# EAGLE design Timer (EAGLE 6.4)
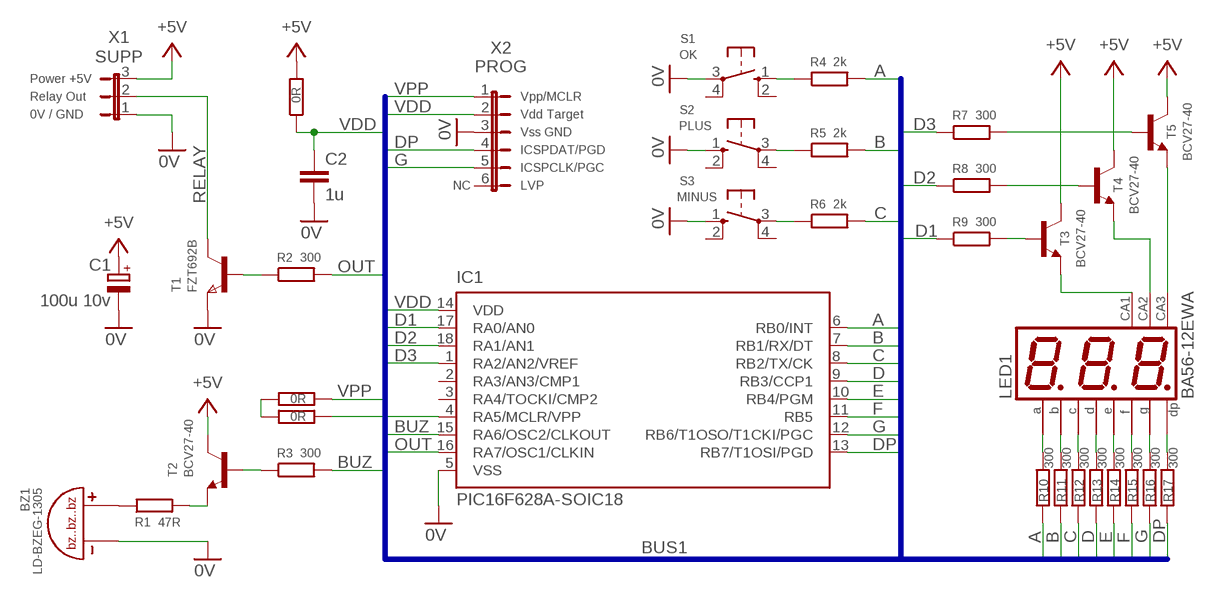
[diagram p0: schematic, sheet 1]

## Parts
BZ1  LD-BZEG-1305  LD-BZEG-1305LOUDITY  [LD-BZEG-1305]
C1  100u 10v  CPOL-EUSMCD  [SMC_D]
C2  1u  C-EUC1206K  [C1206K]
IC1  PIC16F628A-SOIC18  PIC16F628SO  [SO-18W]
J1  0R  R-EU_1206  [RESC3216X71N]
J2  0R  R-EU_1206  [RESC3216X71N]
J3  0R  R-EU_1206  [RESC3216X71N]
LED1  BA56-12EWA  [BX56-12]
R1  47R  R-EU_1206  [RESC3216X71N]
R2  300  R-EU_1206  [RESC3216X71N]
R3  300  R-EU_1206  [RESC3216X71N]
R4  2k  R-EU_1206  [RESC3216X71N]
R5  2k  R-EU_1206  [RESC3216X71N]
R6  2k  R-EU_1206  [RESC3216X71N]
R7  300  R-EU_1206  [RESC3216X71N]
R8  300  R-EU_1206  [RESC3216X71N]
R9  300  R-EU_1206  [RESC3216X71N]
R10  300  R-EU_1206  [RESC3216X71N]
R11  300  R-EU_1206  [RESC3216X71N]
R12  300  R-EU_1206  [RESC3216X71N]
R13  300  R-EU_1206  [RESC3216X71N]
R14  300  R-EU_1206  [RESC3216X71N]
R15  300  R-EU_1206  [RESC3216X71N]
R16  300  R-EU_1206  [RESC3216X71N]
R17  300  R-EU_1206  [RESC3216X71N]
S1  OK  10-XX  [B3F-10XX]
S2  PLUS  10-XX  [B3F-10XX]
S3  MINUS  10-XX  [B3F-10XX]
T1  FZT692B  NPNSOT223  [SOT223]
T2  BCV27-40  -NPN-SOT23_BEC  [SOT23-EBC]
T3  BCV27-40  -NPN-SOT23_BEC  [SOT23-EBC]
T4  BCV27-40  -NPN-SOT23_BEC  [SOT23-EBC]
T5  BCV27-40  -NPN-SOT23_BEC  [SOT23-EBC]
X1  SUPP  JP2W  [JP2W]
X2  PROG  JP6W  [JP6W]

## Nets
0V: BZ1.P$2 C1.- C2.2 IC1.5(VSS) S1.3(P) S2.1(S) S3.1(S) T1.3(E) X1.1 X2.3
+5V: C1.+ J1.2 T2.C T3.C T4.C T5.C X1.3
A: IC1.6(RB0/INT) R4.2 R10.1
B: IC1.7(RB1/RX/DT) R5.2 R11.1
BUZ: IC1.15(RA6/OSC2/CLKOUT) R3.2
C: IC1.8(RB2/TX/CK) R6.2 R12.1
D: IC1.9(RB3/CCP1) R13.1
D1: IC1.17(RA0/AN0) R9.1
D2: IC1.18(RA1/AN1) R8.1
D3: IC1.1(RA2/AN2/VREF) R7.1
DP: IC1.13(RB7/T1OSI/PGD) R17.1 X2.4
E: IC1.10(RB4/PGM) R14.1
F: IC1.11(RB5) R15.1
G: IC1.12(RB6/T1OSO/T1CKI/PGC) R16.1 X2.5
N$1: LED1.11(A) R10.2
N$2: LED1.7(B) R11.2
N$3: LED1.4(C) R12.2
N$4: LED1.2(D) R13.2
N$5: LED1.1(E) R14.2
N$6: LED1.10(F) R15.2
N$7: LED1.5(G) R16.2
N$8: LED1.3(DP) R17.2
N$9: LED1.12(CA) T3.B(E)
N$10: LED1.9(CA) T4.B(E)
N$11: LED1.8(CA) T5.B(E)
N$12: R9.2 T3.E(B)
N$13: R8.2 T4.E(B)
N$14: R7.2 T5.E(B)
N$15: R4.1 S1.1(S)
N$16: R5.1 S2.3(P)
N$17: R6.1 S3.3(P)
N$18: R2.1 T1.1(B)
N$19: R3.1 T2.E(B)
N$20: BZ1.P$1 R1.1
N$21: R1.2 T2.B(E)
N$23: J2.1 J3.1
OUT: IC1.16(RA7/OSC1/CLKIN) R2.2
RELAY: T1.2(C) T1.4(C) X1.2
VDD: C2.1 IC1.14(VDD) J1.1 X2.2
VPP: J3.2 X2.1
VPP': IC1.4(RA5/MCLR/VPP) J2.2
Unconnected: IC1.2(RA3/AN3/CMP1) IC1.3(RA4/TOCKI/CMP2) S1.2(S1) S1.4(P1) S2.2(S1) S2.4(P1) S3.2(S1) S3.4(P1) X2.6

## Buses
BUS1

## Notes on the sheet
- Power +5V
- Relay Out | Vpp/MCLR
- 0V / GND | Vdd Target
- Vss GND
- ICSPDAT/PGD
- ICSPCLK/PGC
- NC | LVP

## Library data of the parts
BZ1 = Timer:LD-BZEG-1305
C1 = Timer:CPOL-EU: POLARIZED CAPACITOR, European symbol
C2 = Timer:C-EU: CAPACITOR, European symbol
IC1 = Timer:PIC16F62*: FLASH-Based 8-Bit CMOS Microcontroller Source: http://ww1.microchip.com/downloads/en/DeviceDoc/40300C.pdf; MF: MICROCHIP; MPN: PIC16F628-20I/SO; OC_FARNELL: 9760415; OC_NEWARK: 23C4986
J1-J3 R1-R17 = Timer:R-EU_: RESISTOR, European symbol
LED1 = Timer:B?56-12*WA: 14.22mm (0.56INCH) THREE DIGIT NUMERIC DISPLAY Source: http://www.kingbright.com .. BA56-11EWA(Ver1189474895.pdf; OC_FARNELL: unknown; OC_NEWARK: unknown
S1-S3 = Timer:10-XX: OMRON SWITCH; MPN: B3F-1000; OC_FARNELL: 176432; OC_NEWARK: 36M3542
T1 = Timer:NPNSOT223: NPN TRANSISTOR; MPN: DJT4031N-13; OC_FARNELL: 1710672; OC_NEWARK: 25R4490
T2-T5 = Timer:*-NPN-: NPN Transistror
X1 = Timer:JP2W: JUMPER
X2 = Timer:JP6W

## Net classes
0 default: width 0.305 mm, drill 0.508 mm, clearance 0.305 mm

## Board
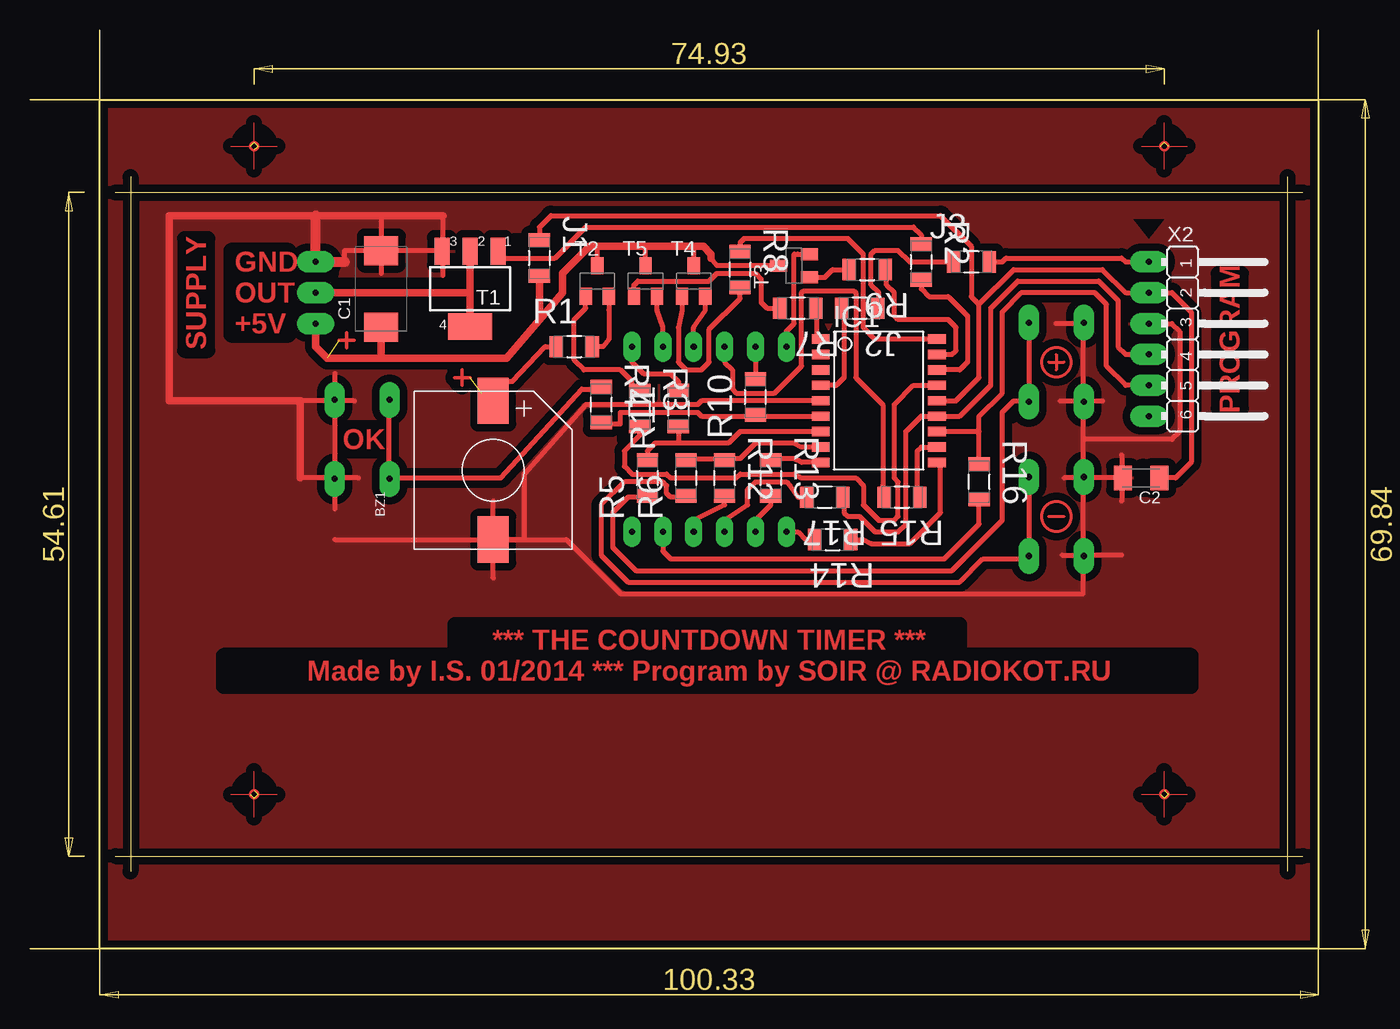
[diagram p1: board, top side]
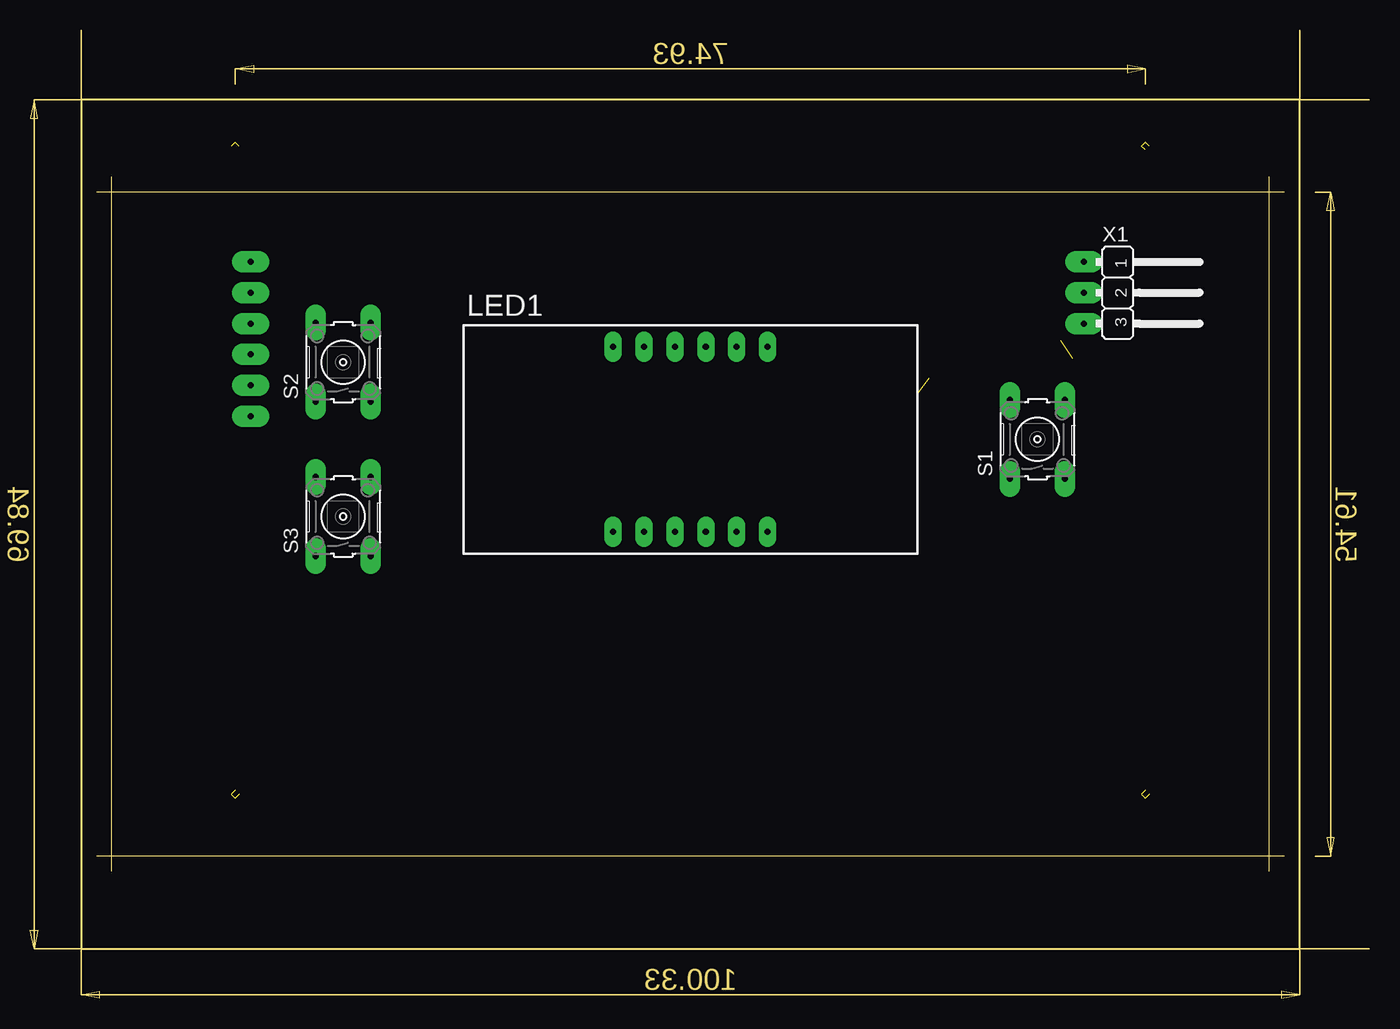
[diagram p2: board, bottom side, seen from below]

Size 110.21 x 79.67 mm. Coordinates in mm from the lower left corner, seen from the top.
Outline: 103.5,10.46 103.5,67.61
Outline: 8.25,67.61 8.25,10.46
Outline: 6.98,11.73 104.75,11.73
Outline: 6.98,66.34 104.75,66.34
Outline: 5.71,4.11 5.71,73.96 106.05,73.96 106.05,4.11 5.71,4.11
Copper layers (1*2): Top 0.035mm / dielectric 1.5mm / Route2 0.035mm
Design rules "default *": minimum track width 12mil, minimum drill 20mil, track to track 12mil, track to pad 12mil, pad to pad 12mil, via to via 12mil, smd to smd 12mil, copper to edge 20mil, drill to drill 40mil, minimum pad ring 10mil, minimum via ring 8mil, stop-mask expansion 6mil, vias tented up to drill 0mil, thermal gap 24mil
tRestrict: area 50.5,37.1 to 51.1,39.7; area 53,37.1 to 53.7,39.7; area 55.6,37.1 to 56.2,39.7; area 58.1,37.1 to 58.7,39.7; area 60.6,37.1 to 61.3,39.7; area 60.6,52.4 to 61.3,54.9; area 58.1,52.4 to 58.7,54.9; area 55.6,52.4 to 56.2,54.9; area 53,52.4 to 53.7,54.9; area 50.5,52.4 to 51.1,54.9; area 90.8,48.9 to 93.3,49.5; area 90.8,51.4 to 93.3,52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

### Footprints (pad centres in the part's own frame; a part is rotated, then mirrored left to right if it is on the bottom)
LD-BZEG-1305 = smd 2.54 x 3.81: P$1 0,5.715; P$2 0,-5.715
SMC_D = smd 2.4 x 2.8: + -3.15,0; - 3.15,0
C1206K = smd 1.5 x 2: 1 -1.5,0; 2 1.5,0
SO-18W = smd 0.762 x 1.46: 1 -5.08,-4.788; 2 -3.81,-4.788; 3 -2.54,-4.788; 4 -1.27,-4.788; 5 0,-4.788; 6 1.27,-4.788; 7 2.54,-4.788; 8 3.81,-4.788; 9 5.08,-4.788; 10 5.08,4.788; 11 3.81,4.788; 12 2.54,4.788; 13 1.27,4.788; 14 0,4.788; 15 -1.27,4.788; 16 -2.54,4.788; 17 -3.81,4.788; 18 -5.08,4.788
RESC3216X71N = smd 1.118 x 1.753: 1 -1.473,0; 2 1.473,0
BX56-12 = drill 0.5 pad 1.422 long: 1 -6.35,-7.62; 2 -3.81,-7.62; 3 -1.27,-7.62; 4 1.27,-7.62; 5 3.81,-7.62; 6 6.35,-7.62; 7 6.35,7.62; 8 3.81,7.62; 9 1.27,7.62; 10 -1.27,7.62; 11 -3.81,7.62; 12 -6.35,7.62
B3F-10XX = drill 0.5 pad 1.7 long: 1 -3.251,2.261; 2 3.251,2.261; 3 -3.251,-2.261; 4 3.251,-2.261
SOT223 = smd 1.219 x 2.235: 1 -2.311,-3.099; 2 0,-3.099; 3 2.311,-3.099 | smd 3.6 x 2.2: 4 0,3.099
SOT23-EBC = smd 1 x 1.4: B 0.95,-1.259; C 0,1.259; E -0.95,-1.259
JP2W = drill 0.5 pad 1.778 long: 1 -2.54,-1.27; 2 0,-1.27; 3 2.54,-1.27
JP6W = drill 0.5 pad 1.778 long: 1 -6.35,-2.54; 2 -3.81,-2.54; 3 -1.27,-2.54; 4 1.27,-2.54; 5 3.81,-2.54; 6 6.35,-2.54

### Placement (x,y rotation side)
BZ1  38.1,43.48 0 top
C1  28.89,58.4 90 top
C2  91.44,42.84 180 top
IC1  69.85,49.19 270 top
J1  41.91,60.94 270 top
J2  68.26,56.81 180 top
J3  77.47,60.62 0 top
LED1  55.88,46.02 0 bottom
R1  44.77,53.64 0 top
R2  73.34,60.62 270 top
R3  50.16,48.56 270 top
R4  46.99,48.87 270 top
R5  50.8,42.84 90 top
R6  53.98,42.84 90 top
R7  63.18,56.81 180 top
R8  58.42,59.99 270 top
R9  68.9,59.99 180 top
R10  59.69,49.51 90 top
R11  53.34,48.56 90 top
R12  57.15,42.84 270 top
R13  60.96,42.84 270 top
R14  66.04,37.76 180 top
R15  71.75,41.25 180 top
R16  78.11,42.52 270 top
R17  65.41,41.25 180 top
S1  27.3,46.02 90 bottom
S2  84.45,52.37 90 bottom
S3  84.45,39.67 90 bottom
T1  36.2,58.4 180 top
T2  46.67,59.03 0 top
T3  62.87,60.3 90 top
T4  54.61,59.03 0 top
T5  50.64,59.03 0 top
X1  22.23,58.08 270 bottom
X2  94.61,54.27 270 top

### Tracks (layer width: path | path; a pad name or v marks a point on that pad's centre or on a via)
0V
  Top 0.406: BZ1.P$2 44.13,37.76 48.58,33.32 86.68,33.32 86.68,36.49 | T1.3 33.66,61.66 33.66,61.89 | IC1.5 55.25,49.19 54.93,48.87 45.72,48.87 40.64,43.16 40.64,37.76 BZ1.P$2 | 86.68,55.86 86.68,49.19 86.68,46.02 | 33.97,62.21 33.97,64.43 | 86.68,36.49 86.68,42.84 | 86.68,42.84 86.68,46.02 | S2.1 86.64,49.19 | 86.64,36.49 S3.1 87.24,36.41 87.31,36.49 89.85,36.49 | 25.08,37.76 BZ1.P$2 | 26.67,49.19 22.23,49.19 | 26.99,42.84 22.23,42.84 | 25.08,40.3 25.08,51.41 | 38.1,34.59 38.1,40.94 | 33.97,59.51 33.97,61.41 | 84.93,36.49 86.68,36.49 | 84.77,49.19 86.52,49.19 | X2.3 93.98,55.54 94.61,54.91 94.61,46.65 93.98,46.02 86.68,46.02 | C2.2 86.68,42.84 | 86.68,42.84 85.09,42.84 | 89.85,44.75 89.85,40.94 | 87,55.54 84.45,55.54 | 87,49.19 88.27,49.19 | 25.88,60.62 25.88,61.57 28.89,61.57 | 28.89,61.57 C1.- 28.89,59.67 | 28.73,64.43 28.89,64.43 28.89,61.57 | 28.89,61.57 33.97,61.57
  Top 0.61: 33.97,64.43 28.73,64.43 23.49,64.43 11.43,64.43 11.43,49.19 22.23,49.19 22.23,42.84 | 33.66,61.89 33.97,62.21 | 86.64,49.19 86.68,49.19 | 86.64,36.49 86.68,36.49 | S1.3 25.08,42.73
  Top 0.813: 23.49,64.43 X1.1 25.88,60.62
  pour Top (isolate 0.61): 8.89,12.36 8.89,65.7 102.87,65.7 102.87,12.36
0V1  (3 unrouted)
  Top 0.1: 16.51,16.81 18.1,16.81 | 18.41,14.9 18.41,16.49 | 18.73,16.81 20.32,16.81 | 18.41,17.12 18.41,18.71
0V4  (2 unrouted)
  Top 0.1: 91.44,70.15 93.03,70.15 | 93.66,70.15 95.25,70.15 | 93.34,70.46 93.34,72.05
0V6  (3 unrouted)
  Top 0.1: 91.44,16.81 93.03,16.81 | 93.34,14.9 93.34,16.49 | 93.66,16.81 95.25,16.81 | 93.34,17.12 93.34,18.71
0V8  (3 unrouted)
  Top 0.1: 16.51,70.15 18.1,70.15 | 18.41,68.24 18.41,69.83 | 18.73,70.15 20.32,70.15 | 18.41,70.46 18.41,72.05
0V9
  Top 0.1: 93.34,68.24 93.34,69.83
+5V  (1 unrouted)
  Top 0.305: 26.67,54.17 26.04,54.17 | 26.04,54.17 25.4,54.17 | 26.04,54.81 26.04,54.17 | 26.04,54.17 26.04,53.54
  Top 0.406: T3.C 56.52,60.3 56.04,60.94 | 54.61,61.89 T4.C | T5.C 50.64,61.89 | T2.C 46.67,61.89
  Top 0.61: X1.3 23.49,53.64 24.45,52.68 28.89,52.68 | 28.89,52.68 39.21,52.68 41.91,55.86 | 56.04,60.94 56.04,61.26 55.4,61.89 54.61,61.89 50.64,61.89 46.67,61.89 46.04,61.89 43.82,59.67 43.82,58.08 41.91,55.86 | J1.2 41.91,55.86 | C1.+ 28.89,52.68
A
  Top 0.406: R4.2 47.62,47.29 48.58,47.29 48.58,48.24 54.93,48.24 55.25,47.92 59.05,47.92 R10.1 60.33,47.92 IC1.6
B
  Top 0.406: IC1.7 58.42,46.65 57.47,45.7 53.34,45.7 | 53.34,45.7 51.44,45.7 50.8,45.06 R5.2 | R11.1 53.34,45.7
BUZ
  Top 0.406: R3.2 50.16,46.33 48.9,45.06 48.9,43.79 49.53,43.16 52.39,43.16 52.7,42.84 58.1,42.84 58.42,43.16 62.87,43.16 63.5,42.84 67.94,42.84 68.58,42.21 68.58,40.62 69.85,39.35 71.12,39.35 71.44,39.67 71.44,42.52 71.12,42.84 71.12,48.87 72.71,50.46 IC1.15
C
  Top 0.406: IC1.8 63.5,45.38 62.87,45.7 59.69,45.7 58.42,44.43 57.79,44.43 R12.1 56.52,44.43 54.61,44.43 R6.2
D
  Top 0.406: IC1.9 63.5,44.11 62.87,44.43 61.59,44.43 R13.1
D1
  Top 0.406: IC1.17 75.88,53 76.2,53.32 76.2,55.22 75.56,55.86 71.44,55.86 71.12,56.18 71.12,58.08 70.48,58.72 70.48,59.35 R9.1
D2
  Top 0.406: IC1.18 69.53,54.27 68.58,55.22 68.58,61.26 67.31,62.53 58.74,62.53 58.42,62.21 R8.1
D3
  Top 0.406: IC1.1 64.77,54.59 64.77,56.18 R7.1
DP
  Top 0.406: R17.1 66.99,40.62 66.99,39.98 67.31,39.67 68.26,39.67 69.53,38.4 71.44,38.4 72.07,39.03 72.07,46.65 73.34,47.92 IC1.13 76.52,47.92 79.06,50.46 79.06,56.81 81.28,59.03 87.95,59.03 89.53,57.45 89.53,53.64 90.17,53 X2.4
E
  Top 0.406: R14.1 68.58,37.76 69.22,37.44 72.39,37.44 74.93,39.98 74.93,43.79 IC1.10
F
  Top 0.406: R15.1 73.02,42.21 73.02,45.06 73.34,45.38 IC1.11
G
  Top 0.406: 78.11,46.65 IC1.12 | R16.1 78.11,46.65 | 78.11,46.65 78.11,47.92 80.01,49.83 80.01,56.49 81.6,58.08 87.63,58.08 88.58,57.13 88.58,52.05 90.17,50.46 X2.5
N$1
  Top 0.406: LED1.11 R10.2
N$2
  Top 0.406: LED1.7 49.53,52.37 50.48,51.41 52.7,51.41 53.34,50.78 R11.2
N$3
  Top 0.406: LED1.4 54.61,39.35 57.15,40.62 R12.2
N$4
  Top 0.406: LED1.2 59.69,39.35 60.96,40.62 R13.2
N$5
  Top 0.406: LED1.1 63.18,38.4 63.82,37.76 R14.2
N$6
  Top 0.406: LED1.10 57.15,52.37 57.79,51.73 57.79,50.14 58.1,49.83 61.28,49.83 63.5,52.05 63.5,58.08 63.66,58.24 67.79,58.24 67.94,58.08 67.94,51.1 70.17,48.87 70.17,42.21 70.48,41.57 R15.2
N$7
  Top 0.406: LED1.5 52.07,36.81 52.7,36.17 75.25,36.17 78.11,39.03 R16.2
N$8
  Top 0.406: LED1.3 57.15,39.35 59.05,40.62 59.05,41.89 59.69,42.52 62.23,42.52 62.55,42.21 63.18,41.25 R17.2
N$9
  Top 0.406: LED1.12 62.23,54.91 62.87,55.54 62.87,61.26 63.18,61.26 T3.B
N$10
  Top 0.406: LED1.9 54.61,55.22 55.56,56.65 T4.B
N$11
  Top 0.406: LED1.8 52.07,55.22 51.59,56.65 T5.B
N$12
  Top 0.406: T3.E 65.41,59.35 66.04,59.99 R9.2
N$13
  Top 0.406: T4.E 53.66,56.65 53.34,55.22 53.34,52.37 53.98,51.73 55.25,51.73 55.88,52.37 55.88,55.06 58.42,57.6 R8.2
N$14
  Top 0.406: T5.E 49.69,58.72 50.01,59.03 55.88,59.03 56.52,59.67 59.69,59.67 60.17,59.19 60.17,57.29 60.64,56.81 R7.2
N$15
  Top 0.406: S1.1 30.16,42.84 38.73,42.84 45.4,50.14 46.99,50.14 R4.1
N$16
  Top 0.406: R5.1 50.16,41.25 49.21,41.25 47.94,39.98 47.94,37.13 49.85,35.22 75.88,35.22 80.01,39.35 80.01,48.24 80.96,49.19 81.92,49.19 S2.3
N$17
  Top 0.406: R6.1 53.34,41.25 52.7,41.25 52.39,41.57 52.39,42.21 52.07,42.52 48.9,42.52 46.99,40.62 46.99,36.49 49.21,34.27 76.52,34.27 78.42,36.17 81.6,36.17 S3.3
N$18
  Top 0.406: R2.1 73.34,62.84 72.71,63.48 45.72,63.48 43.18,60.94 38.73,60.94 38.73,61.57 T1.1
N$19
  Top 0.406: R3.1 49.53,50.14 49.53,50.78 48.58,51.73 45.56,51.73 44.77,52.52 44.77,55.86 45.72,56.81 T2.E
N$20  (1 unrouted)
  Top 0.305: 34.92,51.1 35.56,51.1 | 35.56,51.1 36.2,51.1 | 35.56,50.46 35.56,51.1 | 35.56,51.1 35.56,51.73
  Top 0.406: BZ1.P$1 38.73,50.78 39.69,50.78 42.39,53.64 R1.1
  Top 0.61: 37.15,49.83 BZ1.P$1
N$21
  Top 0.406: T2.B 47.62,56.65 47.62,54.27 47.15,53.64 R1.2
N$22
  pour Top (isolate 0.025, no thermals): 65.72,54.91 66.04,55.54 65.41,55.54
N$23
  Top 0.406: J2.1 69.85,57.45 69.85,58.08 69.22,58.72 69.22,61.26 69.53,61.57 71.44,61.57 72.39,60.62 J3.1
N$24
  Top 0.406: 29.53,42.68 29.53,49.35
N$28
  Top 0.406: 82.23,49.19 82.23,55.54
N$29
  Top 0.406: 82.23,36.49 82.23,42.84
N$30
  Top 0.254: 83.82,39.67 85.09,39.67
N$31
  Top 0.254: 84.45,52.37 85.09,52.37 | 84.45,53 84.45,52.37 | 84.45,52.37 84.45,51.73 | 83.82,52.37 84.45,52.37
N$34
  cutout Top (isolate 0.025, no thermals): 92.08,62.53 93.34,64.11 90.81,64.11
N$84
  pour Top (isolate 0.61): 103.66,73.64 6.03,73.64 6.03,4.42 105.73,4.42 105.73,73.64 103.82,73.64 103.82,11.41 7.94,11.41 7.94,66.65 103.66,66.65
OUT
  Top 0.406: R2.2 73.34,58.4 73.98,57.76 75.56,57.76 77.15,56.18 77.15,52.37 76.52,51.73 IC1.16
RELAY
  Top 0.61: X1.2 36.2,58.08 | T1.4 36.2,58.08 | 36.2,58.08 T1.2
VDD
  Top 0.406: IC1.14 76.2,49.19 78.11,51.1 78.11,57.13 | 78.11,57.13 80.96,59.99 88.27,59.99 90.17,58.08 X2.2 93.98,58.08 95.57,56.49 95.57,44.11 94.3,42.84 C2.1 | 78.11,57.13 77.47,57.76 77.47,61.89 74.93,64.43 42.86,64.43 41.91,63.48 J1.1
VPP
  Top 0.406: J3.2 80.01,60.62 80.33,60.94 89.85,60.94 90.17,60.62 X2.1
VPP'
  Top 0.406: J2.2 66.99,56.49 66.99,51.1 66.36,50.46 IC1.4
(copper drawn outside any net)
  shapes: Top circle x6

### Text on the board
Top: GND | SUPPLY | OUT | +5V | PROGRAM | OK | *** THE COUNTDOWN TIMER *** | Made by I.S. 01/2014 *** Program by SOIR @ RADIOKOT.RU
